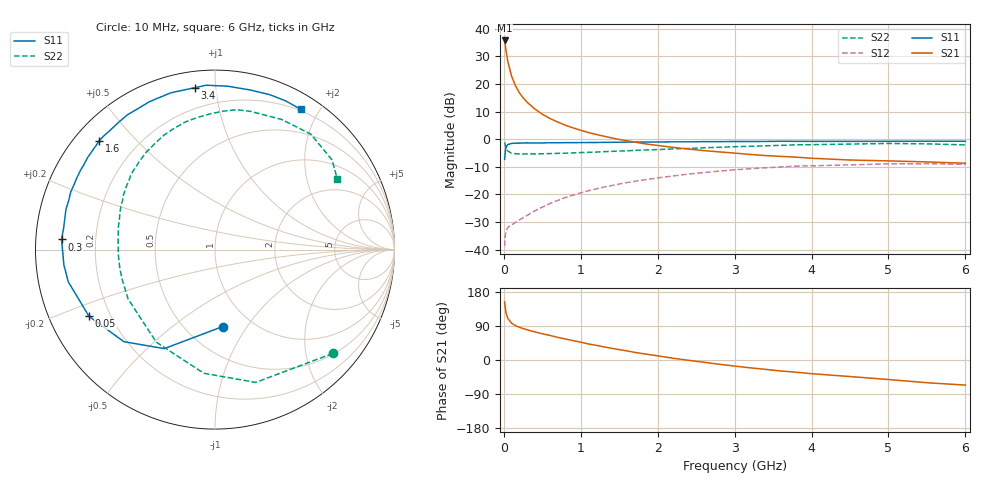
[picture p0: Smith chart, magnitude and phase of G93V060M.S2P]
! SIEMENS Small Signal Semiconductors
! BFG235
! Si NPN RF Bipolar Junction Transistor in SOT223
! VCE = 3 V  IC = 60 mA
! Common Emitter S-Parameters:  July  1994
# GHz  S  MA  R  50
!  f  S11  S21  S12  S22
! GHz  MAG  ANG  MAG  ANG  MAG  ANG  MAG  ANG
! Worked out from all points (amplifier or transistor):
!   40 points, 10 MHz to 6 GHz, reference 50 ohm
!   highest |S21| = 35.8 dB at 10 MHz (marker M1)
!   |S21| within 3 dB of that: start of sweep to 25.16 MHz
!   unconditionally stable (mu >= 1): 485.2 MHz to 1.441 GHz
!   at 200 MHz: K = 0.71, MSG = 23.1 dB, |S12| = -29.3 dB
!   at 1.5 GHz: K = 0.99, MSG = 8.1 dB, |S12| = -16.3 dB
!   at 6 GHz: K = 0.93, MSG = 0.2 dB, |S12| = -9.2 dB
!   S11 on the Smith chart (normalised r, x): 10 MHz: 0.74, -0.78; 50 MHz: 0.12, -0.24; 300 MHz: 0.08, +0.03; 1.6 GHz: 0.07, +0.40; 3.4 GHz: 0.08, +0.88; 6 GHz: 0.18, +1.77
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0.01  0.4311 -84.4  61.51 153.7  0.0115 64.9  0.8749 -41.4
0.02  0.6198 -117.1  49.05 135.1  0.0184 50.1  0.7739 -73.0
0.03  0.7217 -134.7  38.94 123.1  0.0219 40.8  0.6916 -95.2
0.05  0.7943 -152.1  26.21 110.1  0.025 31.2  0.6108 -122.4
0.1  0.8369 -167.6  13.91 97.3  0.028 30.4  0.5567 -150.5
0.15  0.8465 -174.3  9.35 90.9  0.0309 35.4  0.5434 -162.2
0.2  0.8475 -178.1  7.002 86.6  0.0344 39.1  0.5406 -168.8
0.25  0.8517 178.8  5.64 83.0  0.0377 43.1  0.5386 -173.3
0.3  0.8567 176.2  4.714 80.0  0.0412 46.0  0.5393 -177.0
0.4  0.8518 171.6  3.548 74.3  0.05 50.0  0.5395 177.9
0.5  0.8552 167.9  2.835 69.2  0.0587 52.1  0.5435 173.7
0.6  0.8601 164.8  2.367 64.8  0.0681 53.2  0.5475 170.0
0.7  0.8599 161.2  2.045 59.8  0.0777 53.5  0.5533 166.7
0.8  0.8656 158.3  1.789 55.5  0.0875 53.0  0.5566 163.5
1.1  0.8698 149.3  1.316 42.3  0.1162 49.6  0.5782 154.8
1.6  0.8851 136.7  0.936 24.0  0.1631 40.7  0.6149 141.1
2.2  0.8955 123.1  0.711 4.6  0.2155 28.1  0.6652 124.9
3.2  0.9059 101.4  0.529 -20.6  0.2907 4.9  0.7421 97.9
3.4  0.9092 97.0  0.504 -24.7  0.3026 0.0  0.7568 92.1
4.5  0.9107 77.5  0.419 -43.7  0.3422 -25.3  0.8146 62.9
5.5  0.9174 64.5  0.387 -60.0  0.3593 -47.2  0.8216 37.5
6  0.9159 58.6  0.366 -66.2  0.3486 -55.4  0.787 30.0
